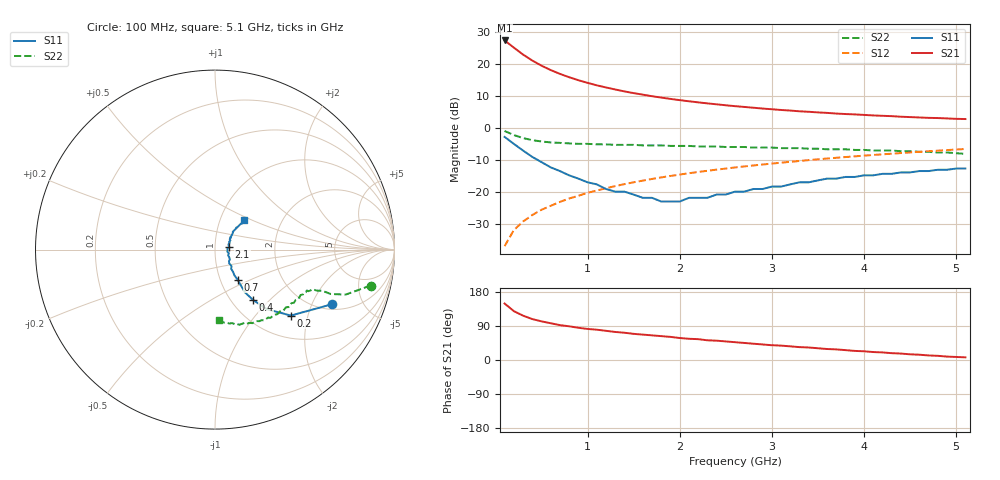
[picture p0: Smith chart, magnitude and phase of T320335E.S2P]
!AT-32033
!S PARAMETERS at Vce=5 V  Ic=10mA.  LAST UPDATED 01-05-95
# ghz s ma r 50
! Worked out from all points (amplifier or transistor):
!   51 points, 100 MHz to 5.1 GHz, reference 50 ohm
!   highest |S21| = 27.3 dB at 100 MHz (marker M1)
!   |S21| within 3 dB of that: start of sweep to 235 MHz
!   unconditionally stable (mu >= 1): 1.061 GHz to 2.362 GHz; 2.454 GHz to 2.533 GHz
!   at 900 MHz: K = 0.99, MSG = 18.1 dB, |S12| = -21.3 dB
!   at 2.6 GHz: K = 1.00, MSG = 9.6 dB, |S12| = -12.4 dB
!   at 5.1 GHz: K = 0.93, MSG = 4.7 dB, |S12| = -6.7 dB
!   S11 on the Smith chart (normalised r, x): 100 MHz: 2.26, -2.85; 200 MHz: 1.47, -1.57; 400 MHz: 1.25, -0.80; 700 MHz: 1.21, -0.42; 2.1 GHz: 1.17, +0.04; 5.1 GHz: 1.30, +0.45
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0.1  0.72 -25.0  23.29 149.0  0.014 78.0  0.89 -13.0
0.2  0.56 -41.0  18 129.0  0.025 73.0  0.77 -19.0
0.3  0.44 -49.0  14.01 117.0  0.034 72.0  0.69 -21.0
0.4  0.35 -53.0  11.29 108.0  0.043 72.0  0.64 -21.0
0.5  0.29 -55.0  9.39 102.0  0.052 72.0  0.61 -22.0
0.6  0.24 -54.0  8.01 97.0  0.06 72.0  0.59 -22.0
0.7  0.21 -53.0  6.98 92.0  0.069 72.0  0.58 -23.0
0.8  0.18 -53.0  6.19 89.0  0.078 72.0  0.57 -24.0
0.9  0.16 -51.0  5.56 85.0  0.086 72.0  0.56 -24.0
1  0.14 -50.0  5.05 82.0  0.096 71.0  0.56 -25.0
1.2  0.11 -44.0  4.28 77.0  0.113 70.0  0.55 -27.0
1.3  0.1 -39.0  3.98 74.0  0.122 70.0  0.54 -28.0
1.4  0.1 -34.0  3.71 72.0  0.131 69.0  0.54 -29.0
1.5  0.09 -28.0  3.49 69.0  0.14 68.0  0.54 -31.0
1.8  0.07 -10.0  2.97 63.0  0.167 66.0  0.53 -34.0
2.1  0.08 11.0  2.6 56.0  0.194 63.0  0.52 -38.0
2.3  0.08 21.0  2.41 52.0  0.212 61.0  0.51 -41.0
2.6  0.1 31.0  2.18 47.0  0.239 58.0  0.5 -45.0
3  0.12 40.0  1.95 39.0  0.275 54.0  0.49 -51.0
3.5  0.15 45.0  1.74 31.0  0.321 49.0  0.47 -58.0
4.3  0.19 45.0  1.52 18.0  0.393 41.0  0.44 -72.0
5.1  0.23 45.0  1.37 7.0  0.465 32.0  0.39 -87.0
